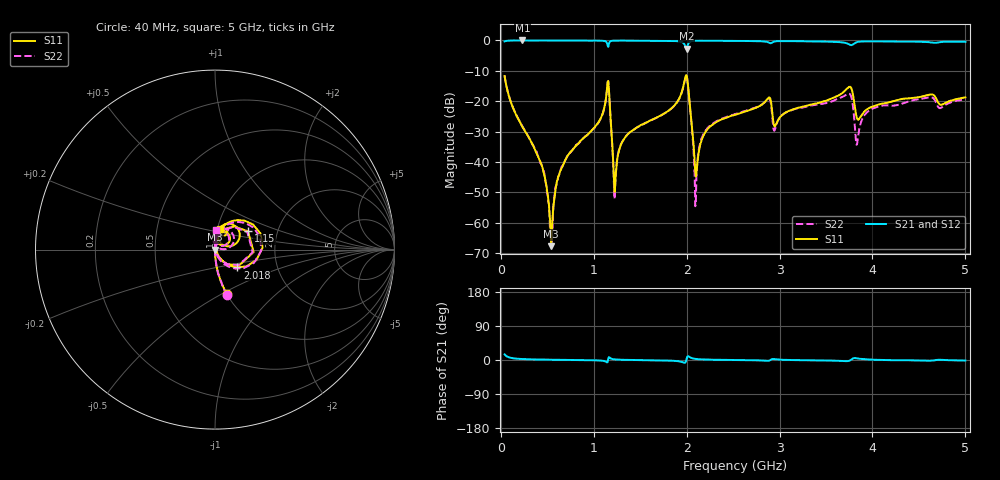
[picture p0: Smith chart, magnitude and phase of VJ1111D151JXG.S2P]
! VJ1111D151JXG
! DATE 02/15/2022  13:14
! CAPACITORS MOUNTED IN SERIES ON 25 MIL THICK MICROSTRIP SUBSTRATE
# GHz  S  MA  R  50.00
!  FREQ  S11M  S11A  S21M  S21A  S12M  S12A  S22M  S22A
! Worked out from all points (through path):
!   801 points, 40 MHz to 5 GHz, reference 50 ohm
!   highest |S21| = 0.00 dB at 232.2 MHz (marker M1); lowest = -2.7 dB at 1.999 GHz (marker M2)
!   lowest |S11| = -67.7 dB at 542.2 MHz (marker M3), VSWR 1.00, Z = 50 + j0.008 ohm
!   |S11| at or under -10 dB: start of sweep to end of sweep
!   |S22| runs from -67.5 to -11.6 dB; largest |S21 - S12| = 0.01
!   S11 on the Smith chart (normalised r, x): 40 MHz: 1.00, -0.54; 1.15 GHz: 1.41, +0.30; 2.018 GHz: 1.26, -0.26; 5 GHz: 1.03, +0.23
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0.04  0.2591 -74.6  0.967 15.0  0.9666 15.0  0.2639 -74.9
0.2322  0.03768 -87.6  0.9996 2.5  0.9993 2.4  0.03844 -87.9
0.4492  0.007983 -87.7  0.9979 1.1  1.001 1.1  0.008051 -87.1
0.5422  0.0004127 11.2  0.9968 0.7  1.001 0.8  0.0005435 16.1
0.6414  0.007217 85.9  0.9975 0.4  0.9996 0.4  0.007349 90.0
0.8708  0.02342 86.5  0.9951 -0.1  0.9997 -0.2  0.02344 87.5
1.1498  0.21 29.0  0.818 -5.1  0.821 -5.1  0.2051 28.5
1.2304  0.004188 50.5  0.993 1.5  0.9973 1.5  0.004248 65.7
1.342  0.0259 87.5  0.9936 0.3  0.9979 0.4  0.026 88.4
1.6954  0.05573 85.7  0.9885 -0.8  0.993 -0.9  0.05564 85.3
1.9992  0.2651 2.3  0.7319 3.6  0.7356 3.5  0.2572 -1.7
2.0178  0.16 -38.5  0.885 9.8  0.8901 9.7  0.1531 -43.6
2.0984  0.005755 8.9  0.9875 2.8  0.9918 2.7  0.002273 75.0
2.2038  0.03155 87.1  0.9883 1.2  0.9932 1.1  0.03309 92.5
2.52  0.05985 85.7  0.9825 -0.1  0.9878 -0.2  0.06153 89.6
2.8796  0.1134 61.6  0.9297 -2.0  0.9338 -2.1  0.1102 62.4
2.954  0.03936 62.7  0.9677 1.9  0.9714 1.8  0.03576 74.7
3.3508  0.08888 83.5  0.9673 -0.8  0.9708 -0.9  0.08556 87.8
3.7476  0.1721 52.2  0.8631 -2.3  0.8674 -2.4  0.1332 48.1
3.8344  0.0518 33.3  0.9398 4.2  0.9445 4.1  0.01994 66.5
4.1754  0.09595 78.8  0.9625 -0.3  0.9692 -0.5  0.08494 89.4
5  0.1159 76.2  0.9493 -1.4  0.9543 -1.6  0.108 87.5
